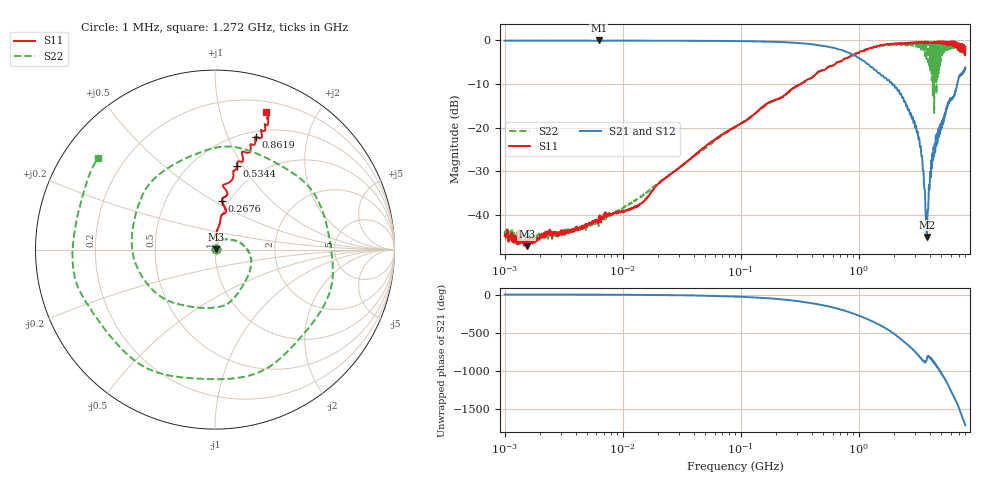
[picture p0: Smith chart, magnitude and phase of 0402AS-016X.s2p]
!s-Parameter Generated by FASTRON Sdn. Bhd.
!FASTRON P/N : 0402AS-016X
!Keysight Technologies: E5071C_MY46733604_B.14.02
!Date: Mon Dec 01 10:31:32 2025
!Version  :Rev00  Mon Dec 01 10:31:32 2025
!Data & Calibration Information:
!Freq  S11:SOLT2(ON)  S21:SOLT2(ON)  S12:SOLT2(ON)  S22:SOLT2(ON)
!PortZ  Port1:50+j0  Port2:50+j0
!When reading reference impedance value at option line is always used.
! Remarks : This data is being provided solely for informational purposes.
# Hz S dB R 50
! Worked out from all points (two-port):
!   1601 points, 1 MHz to 8 GHz, reference 50 ohm
!   highest |S21| = -0.01 dB at 6.268 MHz (marker M1); lowest = -45.0 dB at 3.771 GHz (marker M2)
!   |S21| within 3 dB of the highest: start of sweep to 850.4 MHz
!   lowest |S11| = -47.1 dB at 1.541 MHz (marker M3), VSWR 1.01, Z = 50.4 + j0.189 ohm
!   |S11| at or under -10 dB: start of sweep to 318.8 MHz
!   |S22| runs from -46.0 to -0.1 dB; largest |S21 - S12| = 0.021
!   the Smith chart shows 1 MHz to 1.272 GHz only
!   S11 on the Smith chart (normalised r, x): 1 MHz: 1.01, +0.00; 267.6 MHz: 0.93, +0.55; 534.4 MHz: 0.78, +0.94; 861.9 MHz: 0.56, +1.27; 1.272 GHz: 0.30, +1.39
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1000000  -44.80 18.3  -0.07 -0.3  -0.05 -0.3  -43.70 16.8
1541011  -47.10 25.1  -0.05 -0.5  -0.04 -0.4  -44.70 8.3
4479405  -42.70 42.4  -0.06 -1.4  -0.04 -1.4  -43.10 46.7
6268472  -40.50 39.4  -0.01 -1.6  -0.07 -2.5  -42.50 48.6
2.00676e7  -32.80 66.8  -0.07 -5.9  -0.07 -5.9  -32.70 68.7
8.994653e7  -19.70 84.2  -0.15 -26.1  -0.14 -26.0  -19.90 32.8
2.676115e8  -11.20 81.7  -0.49 -76.4  -0.49 -76.3  -11.40 -59.6
4.006501e8  -8.55 79.9  -0.87 -114.0  -0.86 -114.0  -8.39 -130.0
5.344419e8  -6.33 75.3  -1.38 -150.0  -1.38 -150.0  -6.45 162.0
8.618919e8  -3.50 70.1  -3.10 121.0  -3.08 121.0  -3.54 -9.3
1.052804e9  -2.46 68.4  -4.40 70.6  -4.40 70.5  -2.57 -109.0
1.272209e9  -1.77 69.8  -6.12 17.1  -6.12 17.0  -1.65 142.0
1.550632e9  -1.10 74.4  -8.02 -49.1  -8.03 -49.3  -1.11 4.1
1.7949e9  -0.87 79.4  -9.06 -107.0  -9.07 -107.0  -1.09 -115.0
2.093169e9  -0.70 85.3  -10.80 -179.0  -10.80 -179.0  -1.08 93.7
2.457552e9  -0.76 89.7  -13.90 95.6  -13.90 95.6  -0.74 -80.8
2.824359e9  -0.62 98.3  -18.00 13.5  -17.90 13.3  -0.43 102.0
3.183204e9  -0.42 107.0  -22.00 -73.9  -22.00 -74.2  -1.21 -88.7
3.771001e9  -0.34 119.0  -45.00 -122.0  -45.00 -124.0  -2.75 -37.0
4.115571e9  -0.67 127.0  -27.40 -125.0  -27.40 -125.0  -1.19 -158.0
5.304358e9  -0.80 166.0  -17.80 -13.6  -17.90 -13.9  -0.74 -4.5
8e9  -1.48 -110.0  -6.49 88.3  -6.52 87.9  -3.25 123.0
